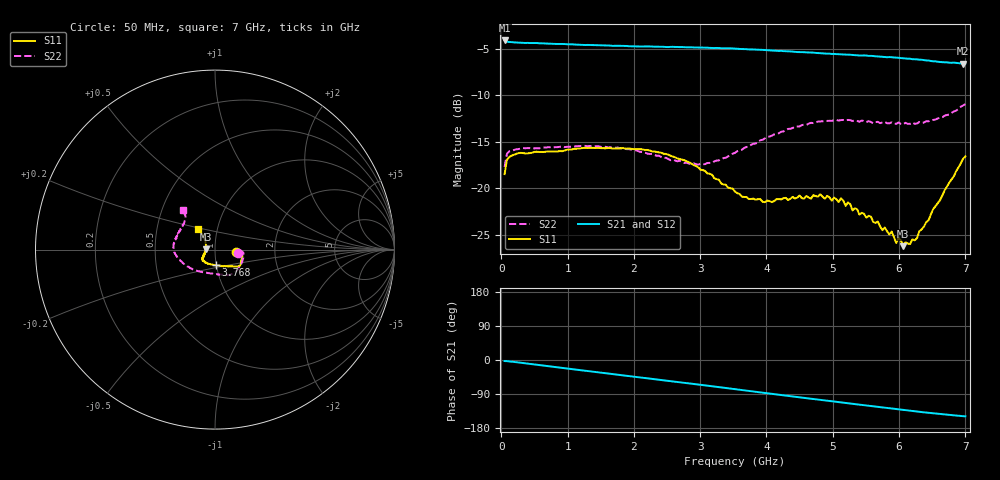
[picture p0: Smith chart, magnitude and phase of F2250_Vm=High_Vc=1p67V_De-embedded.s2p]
! Integrated Device Technology
! Corporate Headquarters
! 6024 Silver Creek Valley Road
! San Jose, CA 95138  USA
! Phone:  1-408-284-8200
! Toll Free:  1-800-223-1366
! Webpage:  http://www.idt.com/
! Timing and RF Division
! 515 Groton Road, Suite 102
! Westford, MA 01886-6024
! Device:  F2250
! Description: Voltage Variable RF Attenuator
! Frequency:  50.0 -  6000.00 MHz
! Package:  3x3 mm Thin QFN Plastic Package: 16 pin
! Ports:  2 RF, 3 DC
!  Pin  1  = GND
!  Pin  2  = NC
!  Pin  3  = RF1  = Port 1
!  Pin  4  = NC
!  Pin  5  = GND
!  Pin  6  = GND
!  Pin  7  = GND
!  Pin  8  = GND
!  Pin  9  = NC
!  Pin 10  = RF2  = Port 2
!  Pin 11  = NC
!  Pin 12  = GND
!  Pin 13  = GND
!  Pin 14  = VCNTRL
!  Pin 15  = VDD
!  Pin 16  = VMODE
! Vcntrl:  1.670 Volts
! Vmode:  +3.300 Volts
! Vdd:  +3.30  Volts
! Current:  1.326 mA
! Data:  The device was measured on a the F2250 evaluation board which has
!  individual transmission lines to the RF pins.  Data was collected
!  using a calibrated network analyzer.  The evaluation board was
!  de-embedded using a TRL calibration technique.
!  The reference plane is the edge of the package pin.
! Misc:  SN 10
!  Action Tracker AT0258
! Date Measured:  2014-11-26
! Date:  2015-10-15  MJV
! Note:
!  Integrated Device Technology supplies this data as a sample of measured
!  data at the package pin for this product.  Your particular data for this
!  product may vary.
!  Data was taken at 25 degrees C.
!  Integrated Device Technology reserves the right to change this data at anytime.
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# GHz S dB R 50
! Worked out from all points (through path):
!   201 points, 50 MHz to 7 GHz, reference 50 ohm
!   highest |S21| = -4.09 dB at 50 MHz (marker M1); lowest = -6.6 dB at 6.965 GHz (marker M2)
!   group delay of S21, straight-line fit = 59.7 ps
!   lowest |S11| = -26.2 dB at 6.062 GHz (marker M3), VSWR 1.10, Z = 45.4 + j0.15 ohm
!   |S11| at or under -10 dB: start of sweep to end of sweep
!   |S22| runs from -17.7 to -10.9 dB; largest |S21 - S12| = 0.0025
!   S11 on the Smith chart (normalised r, x): 50 MHz: 1.27, -0.04; 3.768 GHz: 0.99, -0.17; 7 GHz: 0.81, +0.19
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0.05  -18.48 -7.5  -4.09 -2.7  -4.08 -2.7  -17.71 -8.0
0.08475  -16.94 -4.9  -4.22 -3.0  -4.21 -3.0  -16.30 -5.9
0.2585  -16.21 -8.0  -4.32 -6.5  -4.34 -6.5  -15.78 -11.5
1.2315  -15.67 -29.0  -4.58 -27.6  -4.58 -27.6  -15.43 -44.1
2.37825  -16.13 -37.2  -4.75 -51.8  -4.78 -51.8  -16.49 -71.2
2.969  -17.74 -45.4  -4.83 -64.7  -4.84 -64.7  -17.45 -97.5
3.525  -20.36 -70.2  -4.97 -77.0  -4.97 -77.1  -16.18 -130.5
3.76825  -21.16 -88.0  -5.05 -82.5  -5.05 -82.5  -15.32 -142.8
4.081  -21.50 -108.2  -5.17 -89.4  -5.19 -89.4  -14.34 -156.1
4.7065  -20.75 -136.3  -5.40 -103.0  -5.42 -103.0  -12.98 -174.8
5.08875  -21.48 -144.9  -5.56 -111.1  -5.57 -111.2  -12.71 175.8
5.1235  -21.08 -145.6  -5.58 -111.9  -5.58 -111.9  -12.66 174.8
5.29725  -22.38 -146.4  -5.65 -115.5  -5.65 -115.6  -12.76 171.2
5.6795  -23.59 -156.8  -5.81 -123.6  -5.81 -123.7  -12.85 161.6
5.85325  -24.98 -166.4  -5.88 -127.2  -5.89 -127.4  -13.01 156.1
5.888  -24.67 -167.4  -5.89 -128.0  -5.89 -128.1  -12.90 156.2
5.9575  -25.91 -173.8  -5.93 -129.4  -5.92 -129.5  -13.06 153.3
5.99225  -25.31 -177.7  -5.95 -130.3  -5.94 -130.4  -12.92 152.9
6.06175  -26.24 178.1  -6.01 -131.6  -5.97 -131.7  -13.12 150.1
6.27025  -25.38 155.2  -6.12 -136.0  -6.13 -136.0  -13.03 143.5
6.96525  -16.82 129.8  -6.58 -148.2  -6.57 -148.3  -11.09 130.1
7  -16.57 129.7  -6.58 -148.7  -6.58 -148.9  -10.93 129.3
